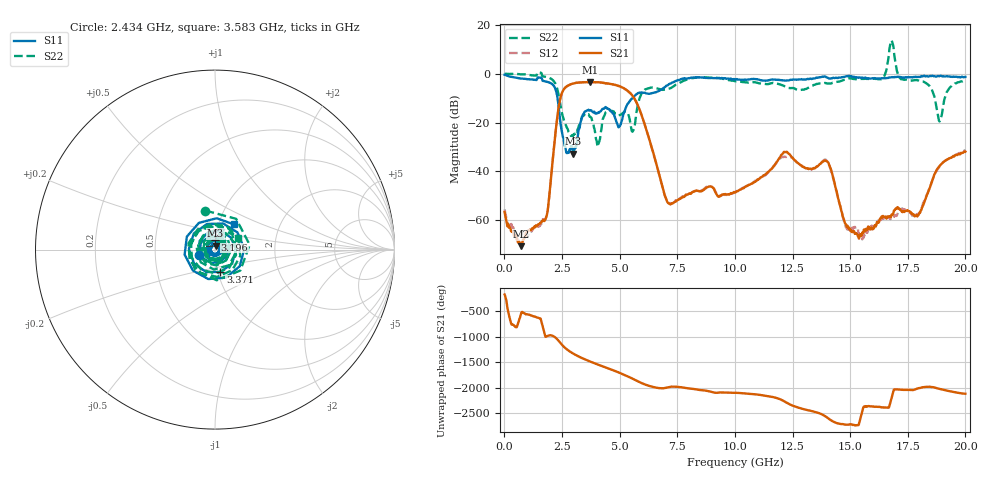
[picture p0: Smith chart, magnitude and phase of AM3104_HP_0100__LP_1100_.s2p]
!Created with skrf (http://scikit-rf.org).
# Hz S RI R 50.0
!freq ReS11 ImS11 ReS21 ImS21 ReS12 ImS12 ReS22 ImS22
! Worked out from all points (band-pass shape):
!   1601 points, 10 MHz to 20 GHz, reference 50 ohm
!   highest |S21| = -3.41 dB at 3.708 GHz (marker M1); lowest = -70.7 dB at 722.1 MHz (marker M2)
!   |S21| within 3 dB of the highest: 2.579 GHz to 5.259 GHz (2.68 GHz wide, 68.4 % of centre)
!   lowest |S11| = -32.7 dB at 2.996 GHz (marker M3), VSWR 1.05, Z = 50.3 + j2.3 ohm
!   |S11| at or under -10 dB: 2.306 GHz to 5.56 GHz (3.254 GHz wide, 82.7 % of centre)
!   |S22| runs from -29.9 to 13.6 dB; largest |S21 - S12| = 0.058
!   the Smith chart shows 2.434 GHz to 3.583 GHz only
!   S11 on the Smith chart (normalised r, x): 2.434 GHz: 0.83, -0.06; 3.196 GHz: 0.99, +0.11; 3.371 GHz: 1.03, -0.26; 3.583 GHz: 1.18, +0.34
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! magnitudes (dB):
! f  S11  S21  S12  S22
! 10 MHz  -0.4  -56.6  -55.6  0.0
! 722.1 MHz  -2.0  -70.7  -66.0  -0.3
! 1.809 GHz  -3.2  -59.0  -58.8  -1.3
! 2.434 GHz  -20.3  -9.9  -9.9  -13.0
! 2.996 GHz  -32.7  -4.0  -4.0  -24.9
! 3.196 GHz  -25.0  -3.6  -3.7  -22.5
! 3.346 GHz  -18.6  -3.5  -3.6  -18.3
! 3.371 GHz  -17.8  -3.5  -3.6  -17.5
! 3.583 GHz  -15.1  -3.4  -3.5  -16.7
! 3.708 GHz  -15.0  -3.4  -3.5  -17.7
! 5.545 GHz  -10.2  -8.8  -8.8  -23.7
! 6.682 GHz  -7.2  -40.1  -40.1  -6.1
! 7.181 GHz  -4.1  -53.5  -53.0  -6.0
! 10.01 GHz  -2.4  -48.7  -48.7  -3.1
! 12.17 GHz  -2.8  -32.1  -34.0  -5.2
! 13.34 GHz  -2.1  -39.1  -39.2  -5.0
! 14.04 GHz  -1.8  -36.3  -36.4  -4.0
! 15.3 GHz  -1.5  -65.6  -63.7  -2.1
! 16.68 GHz  -1.6  -58.5  -58.9  7.3
! 17.95 GHz  -1.3  -58.0  -57.7  -2.7
! 18.89 GHz  -1.0  -37.7  -37.9  -19.5
! 20 GHz  -1.3  -31.9  -31.4  -2.8
